{attribute 'qualified_only'}
VAR_GLOBAL
	bExternalDeviceNotConnected AT %I*	: BOOL;
	bTimeStampUpdateToggle AT %I*		: BOOL;
	DcToExtTimeOffset AT%I* 			: LINT; 
	DcToTcTimeOffset AT%I* 				: LINT; 
	ExtTime AT%I* 						: ULINT; 
	IntTime AT%I* 						: ULINT; 
	EL6688NetId	AT%I*					: T_AmsNetIdArr;
	EL6688SlaveAddr	AT%I*				: UINT;
	bInput AT %I*						: BOOL;
END_VAR
